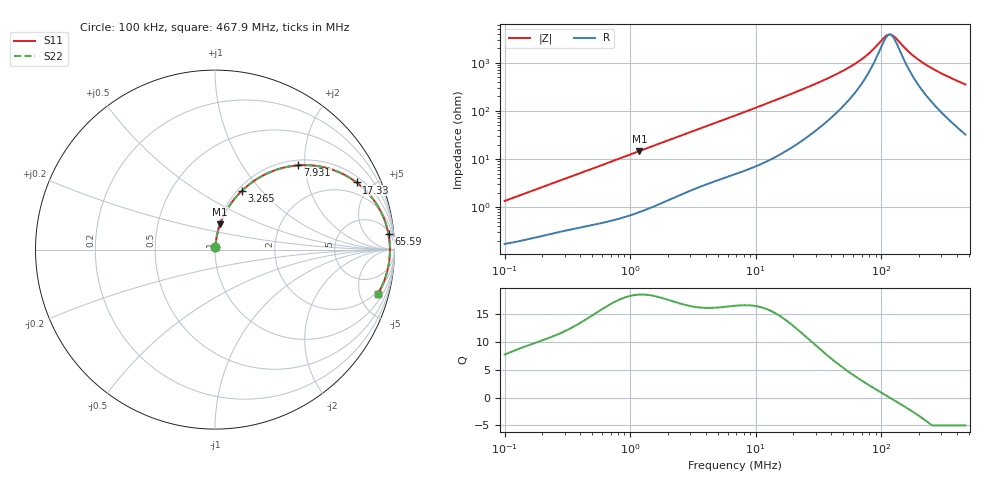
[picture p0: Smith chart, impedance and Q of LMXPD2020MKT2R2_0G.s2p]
! LMXPD2020MKT2R2_0G  S-PARAMETER MODEL  ( General Type )
! Model Generated by TAIYO YUDEN Corporation (https://www.yuden.co.jp/en/)
! Version 1.0
! TAIYO YUDEN Control No. 191023NI43SB-FBB
! Copyright(c) 2019 TAIYO YUDEN CO.,LTD. All Rights Reserved.
! Product Description (link to TY-COMPAS)
! https://ds.yuden.co.jp/TYCOMPAS/or/detail?pn=LMXPD2020MKT2R2M0G&u=M
! Products Name : Inductors
! Characteristics :
!  Inductance : 2.2 uH , SRF(min) : -Hz , DC Resistance(max) : 0.1548 Ohm
!  Rated Current : Saturation :1600 mA , Temp Rise : 1200 mA (40 degC)
!  Case Size : 2.0 x 2.0 / 0.079 x 0.079 [mm/inch] , Thickness : 1.2 / 0.047 [mm/inch]
!  (Conditions: Temperature = 25 degC , DC Bias Current/Voltage = 0A / 0V)
! External Node Assignments :
!  1  o---GGG---o  2
! GND o---------o GND
! Frequency Range : 0.1MHz  -  467.920999MHz  [ 402 STEP ]
# MHz S RI R 50
! Freq[MHz].  S11 Real  S11 Imag  S21 Real  S21 Imag  S12 Real  S12 Imag  S22 Real  S22 Imag
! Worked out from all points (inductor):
!   401 points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, 100 kHz to 467.9 MHz, reference 50 ohm
!   read as one part in series: L = 2.12 uH near 104.3 kHz
!   highest Q = 18.5 at 1.184 MHz (marker M1), where L = 1.97 uH
!   self-resonance near 116.8 MHz
!   S11 on the Smith chart (normalised r, x): 100 kHz: 1.00, +0.03; 3.265 MHz: 1.05, +0.78; 7.931 MHz: 1.11, +1.85; 17.33 MHz: 1.29, +4.05; 65.59 MHz: 7, +20; 467.9 MHz: 1.65, -7.05
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0.1  0.00191 0.0133  0.9981 -0.0133  0.9981 -0.0133  0.00191 0.0133
0.411864  0.00653 0.0518  0.9935 -0.0518  0.9935 -0.0518  0.00653 0.0518
1.184474  0.0284 0.1413  0.9716 -0.1413  0.9716 -0.1413  0.0284 0.1413
1.69632  0.0515 0.1951  0.9485 -0.1951  0.9485 -0.1951  0.0515 0.1951
2.378563  0.09 0.2583  0.91 -0.2583  0.91 -0.2583  0.09 0.2583
3.265474  0.1479 0.3257  0.8521 -0.3257  0.8521 -0.3257  0.1479 0.3257
4.776436  0.2549 0.4059  0.7451 -0.4059  0.7451 -0.4059  0.2549 0.4059
6.986533  0.4057 0.4617  0.5943 -0.4617  0.5943 -0.4617  0.4057 0.4617
7.93075  0.4632 0.4694  0.5368 -0.4694  0.5368 -0.4694  0.4632 0.4694
11.35786  0.6281 0.4534  0.3719 -0.4534  0.3719 -0.4534  0.6281 0.4534
17.33027  0.7884 0.3741  0.2116 -0.3741  0.2116 -0.3741  0.7884 0.3741
28.17346  0.8993 0.2548  0.1007 -0.2548  0.1007 -0.2548  0.8993 0.2548
45.80101  0.9502 0.1493  0.0498 -0.1493  0.0498 -0.1493  0.9502 0.1493
65.59299  0.9667 0.0859  0.0333 -0.0859  0.0333 -0.0859  0.9667 0.0859
82.75365  0.972 0.0498  0.028 -0.0498  0.028 -0.0498  0.972 0.0498
106.6332  0.9746 0.0129  0.0254 -0.0129  0.0254 -0.0129  0.9746 0.0129
116.0364  0.9748 0.000905  0.0252 -0.000905  0.0252 -0.000905  0.9748 0.000905
126.2687  0.9747 -0.0111  0.0253 0.0111  0.0253 0.0111  0.9747 -0.0111
169.7274  0.9719 -0.0543  0.0281 0.0543  0.0281 0.0543  0.9719 -0.0543
218.7041  0.9657 -0.0943  0.0343 0.0943  0.0343 0.0943  0.9657 -0.0943
313.2127  0.948 -0.1597  0.052 0.1597  0.052 0.1597  0.948 -0.1597
467.921  0.9068 -0.2486  0.0932 0.2486  0.0932 0.2486  0.9068 -0.2486
